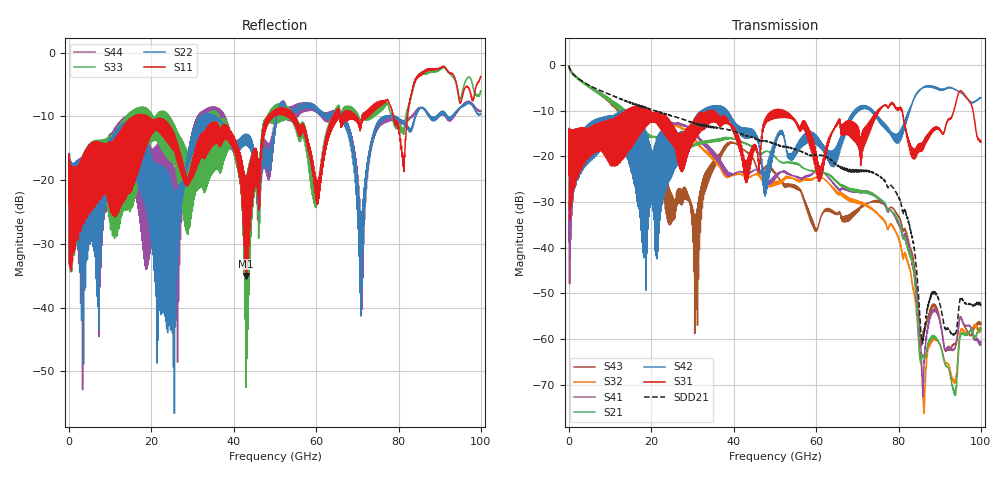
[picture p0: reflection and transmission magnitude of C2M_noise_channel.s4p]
! File created by UCTS
! Freq  S11  S12  S13  S14
!  S21  S22  S23  S24
!  S31  S32  S33  S34
!  S41  S42  S43  S44
# MHz S DB R 50
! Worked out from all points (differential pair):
!   10000 points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, 10 MHz to 100 GHz, reference 50 ohm
!   strongest paths, dB at 10 MHz, 25.01 GHz, 50.01 GHz, 75.01 GHz, 100 GHz:
!     S31: -24.2, -13.0, -10.0, -10.3, -16.9
!     S42: -24.2, -15.5, -17.3, -11.7, -7.2
!     S21: -0.2, -17.4, -20.2, -29.1, -57.9
!     S41: -38.7, -12.9, -24.1, -29.1, -60.6
!     S32: -38.7, -13.3, -25.6, -32.6, -57.5
!     S43: -0.2, -33.8, -23.8, -29.7, -56.5
!   taken as a pair (ports 1,3 in; 2,4 out), SDD21 dB: -0.2, -11.1, -17.2, -24.1, -52.2
!   lowest |S11| = -35.0 dB at 43 GHz (marker M1), VSWR 1.04, Z = 48.4 - j0.61 ohm
!   |S11| at or under -10 dB: start of sweep to 15.85 GHz; 18.95 GHz to 48.23 GHz (29.28 GHz wide, 87.2 % of centre); 54.9 GHz to 64.19 GHz (9.288 GHz wide, 15.6 % of centre)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
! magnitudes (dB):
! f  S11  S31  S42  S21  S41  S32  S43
! 10 MHz  -23.8  -24.2  -24.2  -0.2  -38.7  -38.7  -0.2
! 30.72 GHz  -17.3  -11.7  -12.9  -17.5  -15.1  -16.7  -47.4
! 43 GHz  -35.0  -22.8  -14.0  -17.2  -23.6  -24.4  -19.0
! 70.87 GHz  -11.8  -18.0  -9.7  -27.5  -27.6  -30.0  -31.0
! 78.57 GHz  -9.6  -8.2  -15.3  -32.3  -32.4  -35.2  -31.3
! 86.08 GHz  -2.9  -18.1  -4.9  -63.8  -69.6  -74.5  -58.7
! 100 GHz  -3.7  -16.9  -7.2  -57.9  -60.6  -57.5  -56.5
